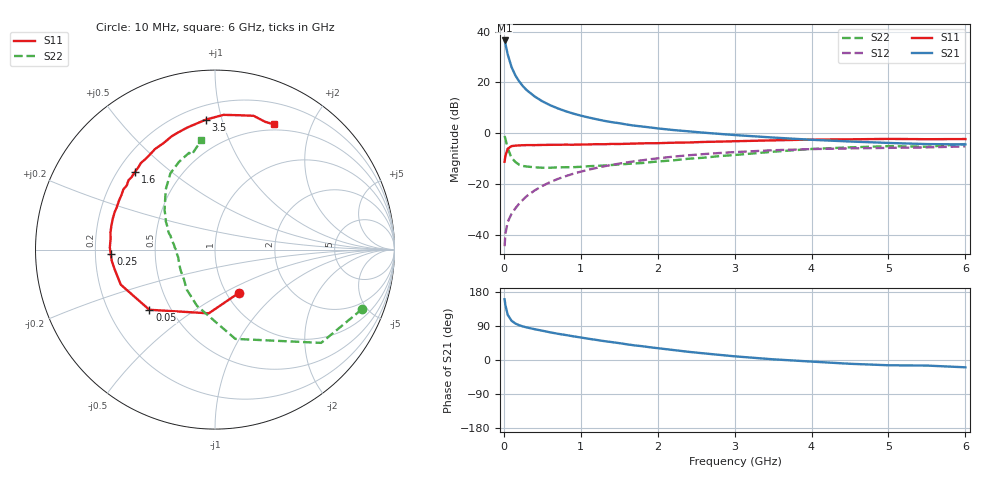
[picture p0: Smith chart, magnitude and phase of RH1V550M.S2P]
! SIEMENS Small Signal Semiconductors
! BFR106
! Si NPN RF Bipolar Junction Transistor in SOT23
! VCE = 1.5 V  IC = 50 mA
! Common Emitter S-Parameters:  August  1996
# GHz  S  MA  R  50
!  f  S11  S21  S12  S22
! GHz  MAG  ANG  MAG  ANG  MAG  ANG  MAG  ANG
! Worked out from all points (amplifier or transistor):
!   36 points, 10 MHz to 6 GHz, reference 50 ohm
!   highest |S21| = 36.5 dB at 10 MHz (marker M1)
!   |S21| within 3 dB of that: start of sweep to 32.59 MHz
!   unconditionally stable (mu >= 1): 219.1 MHz to 2.994 GHz; 4.457 GHz to end of sweep
!   at 250 MHz: K = 1.03, MAG = 21.3 dB, |S12| = -26.1 dB
!   at 1.4 GHz: K = 1.07, MAG = 6.9 dB, |S12| = -12.5 dB
!   at 6 GHz: K = 1.01, MAG = -0.3 dB, |S12| = -5.2 dB
!   S11 on the Smith chart (normalised r, x): 10 MHz: 1.14, -0.60; 50 MHz: 0.38, -0.34; 250 MHz: 0.26, -0.02; 1.6 GHz: 0.27, +0.38; 3.5 GHz: 0.29, +0.89; 6 GHz: 0.43, +1.49
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0.01  0.2756 -61.3  67.2 160.2  0.006 77.6  0.8843 -22.0
0.02  0.3568 -95.6  58.39 145.1  0.0104 67.9  0.7874 -41.3
0.05  0.4961 -137.5  35.83 119.4  0.018 56.8  0.5101 -77.2
0.1  0.5602 -159.6  20.17 103.6  0.026 59.0  0.3291 -107.7
0.15  0.5701 -169.1  13.74 96.2  0.0333 63.1  0.2728 -125.3
0.2  0.5787 -173.8  10.47 91.8  0.0415 66.5  0.2405 -135.9
0.25  0.5819 -177.8  8.377 88.4  0.0496 68.1  0.2272 -145.1
0.3  0.5861 178.9  7.016 85.8  0.0584 69.3  0.2218 -150.7
0.4  0.5847 174.0  5.314 81.3  0.075 70.2  0.214 -159.4
0.5  0.5903 170.7  4.269 77.3  0.0919 69.8  0.21 -165.5
0.6  0.5927 166.6  3.581 73.1  0.1091 69.0  0.2099 -169.2
0.7  0.5952 162.7  3.098 69.3  0.126 68.4  0.213 -172.7
0.9  0.5958 156.6  2.45 62.6  0.1595 65.5  0.2153 -179.0
1.1  0.6031 149.9  2.049 56.1  0.1917 62.4  0.225 177.0
1.3  0.6076 144.0  1.765 50.0  0.2233 59.0  0.2319 172.3
1.6  0.6222 135.7  1.485 41.4  0.2674 53.9  0.2492 166.7
2.2  0.6524 120.8  1.16 26.4  0.3465 43.4  0.2929 154.6
2.8  0.6854 107.0  0.974 13.6  0.4086 33.1  0.3553 142.2
3.5  0.726 94.0  0.825 1.8  0.464 22.1  0.4332 129.3
4.5  0.7605 79.9  0.689 -10.0  0.5041 8.1  0.5285 112.3
5.5  0.7649 68.6  0.613 -14.7  0.5273 -0.3  0.5445 103.8
6  0.7707 64.8  0.605 -19.3  0.5525 -7.0  0.6144 97.1
